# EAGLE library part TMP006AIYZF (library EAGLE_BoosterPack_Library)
TMP006AIYZF This sensor uses a thermopile to absorb the infrared energy emitted from the object being measured and uses the corresponding change in thermopile voltage to determine the object temperature>/p>
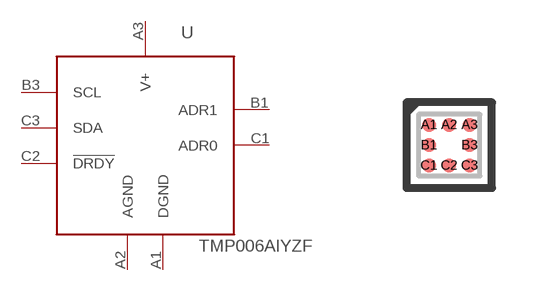
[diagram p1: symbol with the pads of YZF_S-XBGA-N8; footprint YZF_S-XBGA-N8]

Designator prefix U

## TMP006AIYZF  [YZF_S-XBGA-N8]
A1  DGND  pwr
A2  AGND  pwr
A3  V+  pwr
B1  ADR1  in
B3  SCL  in
C1  ADR0  in
C2  !DRDY  out
C3  SDA

## Footprint YZF_S-XBGA-N8 (pad centres in mm)
smd 0.356 x 0.356: A1 -0.508,0.508; A2 0,0.508; A3 0.508,0.508; B1 -0.508,0; B3 0.508,0; C1 -0.508,-0.508; C2 0,-0.508; C3 0.508,-0.508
